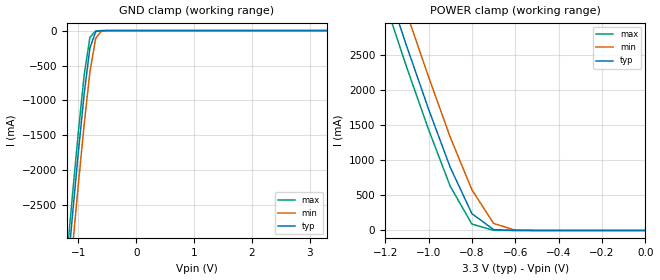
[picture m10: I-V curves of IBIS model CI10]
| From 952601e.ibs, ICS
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|   Model CI10
[Model]   CI10
Model_type   Input
Polarity   Non-Inverting
Enable   Active-High
Vinl =   0.80V
Vinh =   2.00V
C_comp   5.50pF   5.00pF   6.00pF
[Temperature Range]   27.00   70.00   0.000
[Voltage Range]   3.30V   3.10V   3.70V
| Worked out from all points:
|   GND clamp passes 1 mA (typ) near -0.60 V on its own axis
|   POWER clamp passes 1 mA (typ) near -0.61 V on its own axis
[GND_clamp]
| voltage   I(typ)   I(min)   I(max)
-3.3V     -24.05A    -24.49A    -23.79A
-1.2V     -3.55A     -4.02A     -3.26A
-1.1V     -2.63A     -3.1A      -2.34A
-1V       -1.74A     -2.2A      -1.45A
-900mV    -910mA     -1.35A     -640mA
-800mV    -250mA     -590mA     -96.82mA
-700mV    -14.58mA   -110mA     -3.87mA
-600mV    -880uA     -5.82mA    -450uA
-500mV    -88.5uA    -350uA     -45.09uA
3.3V      130pA      8.71nA     110pA
[POWER_clamp]
| voltage   I(typ)   I(min)   I(max)
-3.3V     24.04A     24.47A     23.78A
-1.2V     3.54A      4.01A      3.25A
-1.1V     2.62A      3.09A      2.32A
-1V       1.73A      2.19A      1.44A
-900mV    900mA      1.33A      630mA
-800mV    240mA      580mA      90.95mA
-700mV    12.08mA    100mA      1.95mA
-600mV    280uA      4.78mA     32.65uA
0V        130pA      320pA      130pA
